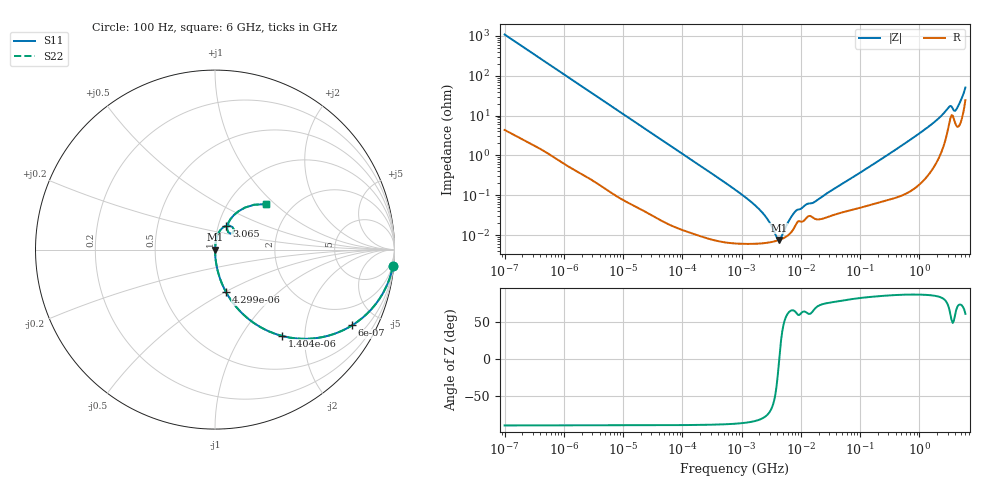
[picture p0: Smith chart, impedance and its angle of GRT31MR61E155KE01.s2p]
!Murata Part Number: GRT31MR61E155KE01
!These Parameters are Measured in Series Mode Connection
!Data Generated on Jun 19, 2026
!  o--ll--o
!Port1  Port2
!  o------o
!Operation Temp=25[degC], DC Bias Voltage=0[V]
!Freq. Start=100[Hz] Stop=6[GHz] 401[Steps]
# Hz S RI R 50
!Freq.(Hz) S11(Real) S11(Imag) S21(Real) S21(Imag) S12(Real) S12(Imag) S22(Real) S22(Imag)
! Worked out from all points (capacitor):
!   401 points, 100 Hz to 6 GHz, reference 50 ohm
!   read as one part in series: C = 1.47 uF near 109 Hz
!   lowest |Z| = 7.61 mohm at 4.246 MHz (marker M1)
!   series resonance near 4.322 MHz, so ESL is about 920 pH
!   S11 on the Smith chart (normalised r, x): 100 Hz: 1, -22; 600 Hz: 1.02, -3.62; 1.404 kHz: 1.01, -1.55; 4.299 kHz: 1.00, -0.51; 3.065 GHz: 1.09, +0.30; 6 GHz: 1.49, +0.88
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100  0.9911 -0.0919  0.00889 0.0919  0.00889 0.0919  0.9911 -0.0919
293  0.9306 -0.2516  0.0694 0.2516  0.0694 0.2516  0.9306 -0.2516
600  0.7648 -0.4213  0.2352 0.4213  0.2352 0.4213  0.7648 -0.4213
1404  0.376 -0.4814  0.624 0.4814  0.624 0.4814  0.376 -0.4814
2008  0.2288 -0.4169  0.7712 0.4169  0.7712 0.4169  0.2288 -0.4169
4299  0.0621 -0.2381  0.9379 0.2381  0.9379 0.2381  0.0621 -0.2381
11009  0.0105 -0.0985  0.9895 0.0985  0.9895 0.0985  0.0105 -0.0985
40335  0.000998 -0.0273  0.999 0.0273  0.999 0.0273  0.000998 -0.0273
774597  6.43e-05 -0.0014  0.9999 0.0014  0.9999 0.0014  6.43e-05 -0.0014
2074311  6.25e-05 -0.000416  0.9999 0.000416  0.9999 0.000416  6.25e-05 -0.000416
2837864  6.57e-05 -0.000225  0.9999 0.000225  0.9999 0.000225  6.57e-05 -0.000225
3712478  7.11e-05 -7.97e-05  0.9999 7.97e-05  0.9999 7.97e-05  7.11e-05 -7.97e-05
4246196  7.55e-05 -9.2e-06  0.9999 9.2e-06  0.9999 9.2e-06  7.55e-05 -9.2e-06
4856642  8.17e-05 6.17e-05  0.9999 -6.17e-05  0.9999 -6.17e-05  8.17e-05 6.17e-05
7947587  0.000166 0.000349  0.9998 -0.000349  0.9998 -0.000349  0.000166 0.000349
1.555665e7  0.000286 0.000574  0.9997 -0.000574  0.9997 -0.000574  0.000286 0.000574
3.124326e8  0.000899 0.011  0.9991 -0.011  0.9991 -0.011  0.000899 0.011
1.431855e9  0.00602 0.0521  0.994 -0.0521  0.994 -0.0521  0.00602 0.0521
3.065283e9  0.0635 0.1323  0.9365 -0.1323  0.9365 -0.1323  0.0635 0.1323
4.193612e9  0.0674 0.1133  0.9326 -0.1133  0.9326 -0.1133  0.0674 0.1133
5.016141e9  0.105 0.1921  0.895 -0.1921  0.895 -0.1921  0.105 0.1921
6e9  0.2859 0.2532  0.7141 -0.2532  0.7141 -0.2532  0.2859 0.2532
